FUNCTION_BLOCK FB_LN_IED_LD1_LLN0 EXTENDS FB_AcsiCommonLogicalNodeClass
VAR_INPUT
	NamPlt: FB_DO_IED_LD1_LLN0_NamPlt := (sClass:='LPL', bLinkResult:=THIS^.AddDataToContainer(ipData:=NamPlt));
	Beh: FB_DO_IED_LD1_LLN0_Beh := (sClass:='ENS', bLinkResult:=THIS^.AddDataToContainer(ipData:=Beh));
	Health: FB_DO_IED_LD1_LLN0_Health := (sClass:='ENS', bLinkResult:=THIS^.AddDataToContainer(ipData:=Health));
	Mod_: FB_DO_IED_LD1_LLN0_Mod := (sObjectName:='Mod', sClass:='ENC', bLinkResult:=THIS^.AddDataToContainer(ipData:=Mod_));
	
	DS1: FB_DS_IED_LD1_LLN0_DS1 := (bLinkResult:=THIS^.AddDataSetToContainer(ipDataSet:=DS1));
	DS2: FB_DS_IED_LD1_LLN0_DS2 := (bLinkResult:=THIS^.AddDataSetToContainer(ipDataSet:=DS2));
	DS3: FB_DS_IED_LD1_LLN0_DS3 := (bLinkResult:=THIS^.AddDataSetToContainer(ipDataSet:=DS3));
	
	urcb101: FB_ScsmUrCBImplClass := (RptID:=(sValue:='IEDLD1/LLN0.urcb101'), DatSet:=(sValue:='IEDLD1/LLN0.DS1'), ConfRev:=(nValue:=1), OptFlds:=(SequenceNumber:=TRUE, ReportTimeStamp:=TRUE, ReasonForInclusion:=TRUE, DataSetName:=TRUE, DataReference:=FALSE, BufferOverflow:=FALSE, EntryID:=FALSE, ConfRevision:=TRUE), TrgOps:=(DataChange:=TRUE, QualityChange:=TRUE, DataUpdate:=TRUE, Integrity:=TRUE, GeneralInterrogation:=TRUE), IntgPd:=(nValue:=5000), bLinkResult:=THIS^.AddUnbufferedReportControlBlockToContainer(ipUnbufferedReportControlBlock:=urcb101));
	brcb101: FB_ScsmBrCBImplClass := (RptID:=(sValue:='IEDLD1/LLN0.brcb101'), DatSet:=(sValue:='IEDLD1/LLN0.DS1'), ConfRev:=(nValue:=1), OptFlds:=(SequenceNumber:=TRUE, ReportTimeStamp:=TRUE, ReasonForInclusion:=TRUE, DataSetName:=TRUE, DataReference:=FALSE, BufferOverflow:=TRUE, EntryID:=TRUE, ConfRevision:=TRUE), TrgOps:=(DataChange:=TRUE, QualityChange:=TRUE, DataUpdate:=TRUE, Integrity:=TRUE, GeneralInterrogation:=TRUE), IntgPd:=(nValue:=5000), bLinkResult:=THIS^.AddBufferedReportControlBlockToContainer(ipBufferedReportControlBlock:=brcb101));
	
	gocb01: FB_GseGoCBImplClass := (GoID:=(sValue:='0001'), DatSet:=(sValue:='IEDLD1/LLN0.DS1'), ConfRev:=(nValue:=1), DstAddress:=(sAddr:='01-0C-CD-01-00-01', nPRIORITY:=4, nVID:=16#000, nAPPID:=16#0001), bLinkResult:=THIS^.AddGooseControlBlockToContainer(ipGooseControlBlock:=gocb01));
	gocb02: FB_GseGoCBImplClass := (GoID:=(sValue:='0002'), DatSet:=(sValue:='IEDLD1/LLN0.DS2'), ConfRev:=(nValue:=1), DstAddress:=(sAddr:='01-0C-CD-01-00-01', nPRIORITY:=4, nVID:=16#000, nAPPID:=16#0002), bLinkResult:=THIS^.AddGooseControlBlockToContainer(ipGooseControlBlock:=gocb02));
	gocb03: FB_GseGoCBImplClass := (GoID:=(sValue:='0003'), DatSet:=(sValue:='IEDLD1/LLN0.DS3'), ConfRev:=(nValue:=1), DstAddress:=(sAddr:='01-0C-CD-01-00-01', nPRIORITY:=4, nVID:=16#000, nAPPID:=16#0003), bLinkResult:=THIS^.AddGooseControlBlockToContainer(ipGooseControlBlock:=gocb03));
END_VAR
VAR
END_VAR

END_FUNCTION_BLOCK
